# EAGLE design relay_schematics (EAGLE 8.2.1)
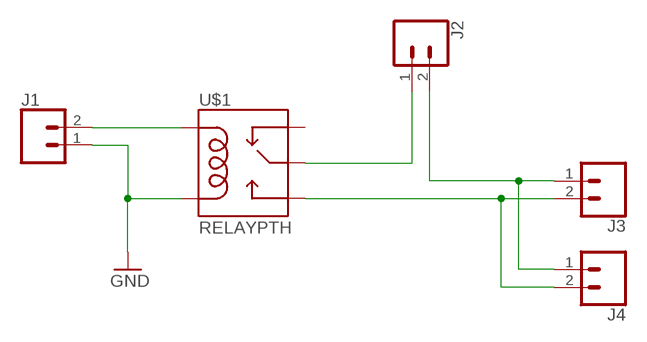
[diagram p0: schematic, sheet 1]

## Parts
J1  CONN_02  [1X02]
J2  CONN_025MM  [SCREWTERMINAL-5MM-2]
J3  CONN_025MM  [SCREWTERMINAL-5MM-2]
J4  CONN_025MM  [SCREWTERMINAL-5MM-2]
U$1  RELAYPTH  [SRD-05VDC-SL-C]

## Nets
GND: J1.1 U$1.COIL0
N$1: J1.2 U$1.COIL1
N$4: J2.1 U$1.SWCOMMON
N$5: J2.2 J3.1 J4.1
N$6: J3.2 J4.2 U$1.SWOPEN
Unconnected: U$1.SWCLOSED(SWCLOSE)

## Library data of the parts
J1 = SparkFun-Connectors:CONN_02: Multi connection point. Often used as Generic Header-pin footprint for 0.1 inch spaced/style header connections
J2-J4 = SparkFun-Connectors:CONN_02: Multi connection point. Often used as Generic Header-pin footprint for 0.1 inch spaced/style header connections; SF_SKU: PRT-08432
U$1 = SRD-05VDC-SL-C:RELAY: SPDT relay (COM-00101)

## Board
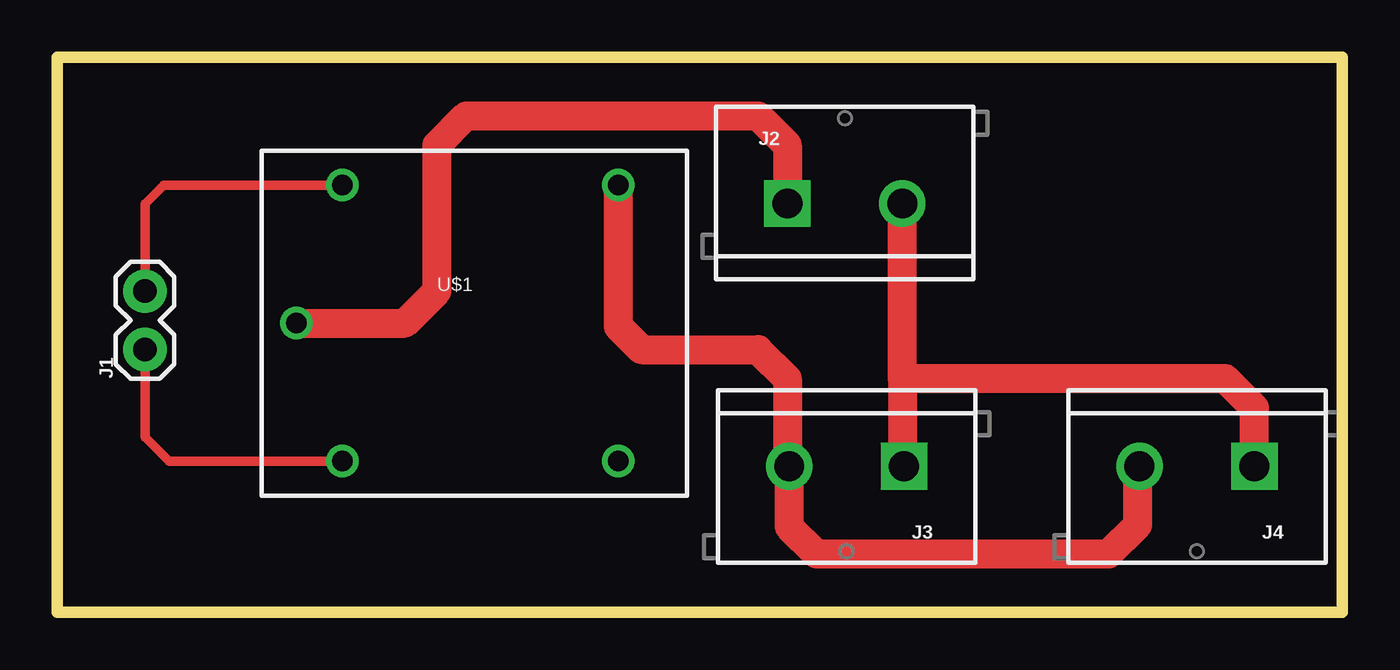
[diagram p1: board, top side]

Size 55.88 x 24.13 mm. Coordinates in mm from the lower left corner, seen from the top.
Outline: 0,24.13 0,0 55.88,0 55.88,24.13 0,24.13
Copper layers (1*16): Top 0.035mm / dielectric 1.5mm / Bottom 0.035mm
Design rules "default": minimum track width 6mil, minimum drill 0.35mm, track to track 6mil, track to pad 6mil, pad to pad 6mil, via to via 6mil, smd to smd 6mil, copper to edge 40mil, drill to drill 6mil, minimum pad ring 10mil, minimum via ring 8mil, stop-mask expansion 4mil, vias tented up to drill 0mil, thermal gap 10mil

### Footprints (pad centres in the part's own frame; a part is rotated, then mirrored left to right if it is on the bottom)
1X02 = drill 1.016 pad 1.88: 1 0,0; 2 2.54,0
SCREWTERMINAL-5MM-2 = drill 1.3 pad 2.032 square: 1 0,0 | drill 1.3 pad 2.032: 2 5,0
SRD-05VDC-SL-C = drill 0.9: COIL0 -5.39,-6.12; COIL1 -5.39,5.88; SWCLOSED 6.61,-6.12; SWCOMMON -7.39,-0.12; SWOPEN 6.61,5.88

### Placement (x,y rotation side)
J1  3.81,11.43 90 top
J2  31.75,17.78 0 top
J3  36.83,6.35 180 top
J4  52.07,6.35 180 top
U$1  17.78,12.7 0 top

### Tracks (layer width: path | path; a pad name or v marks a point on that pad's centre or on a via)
GND
  Top 0.406: U$1.COIL0 4.85,6.58 3.81,7.62 J1.1
N$1
  Top 0.406: U$1.COIL1 4.61,18.58 3.81,17.78 J1.2
N$4
  Top 1.27: U$1.SWCOMMON 15.12,12.58 16.51,13.97 16.51,20.32 17.78,21.59 30.48,21.59 31.75,20.32 J2.1
N$5
  Top 1.27: 36.75,10.16 J2.2 | 36.75,10.16 36.75,6.43 J3.1 | J4.1 52.07,8.89 50.8,10.16 36.75,10.16
N$6
  Top 1.27: J4.2 46.99,6.27 46.99,3.81 45.72,2.54 33.02,2.54 31.83,3.73 J3.2 31.75,6.43 31.75,10.16 30.48,11.43 25.4,11.43 24.39,12.44 U$1.SWOPEN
